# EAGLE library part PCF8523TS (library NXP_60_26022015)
The PCF8523 is a CMOS Real-Time Clock (RTC) and calendar optimized for low power consumption. Data is transferred serially via an I2C-bus with a maximum data rate of 1000 kbit/s. Alarm and timer functions are available with the possibility to generate a wake-up signal on an interrupt pin. An offset register allows fine-tuning of the clock. The PCF8523 has a backup battery switch-over circuit, which detects power failures and automatically switches to the battery supply when a power failure occurs. AAL Eindhoven MK
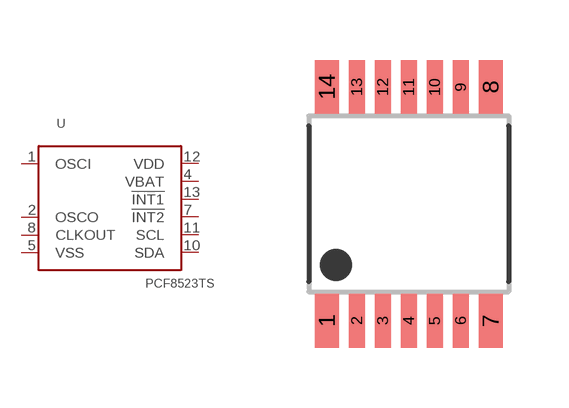
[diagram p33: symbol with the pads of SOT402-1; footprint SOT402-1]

Designator prefix -

## PCF8523TS  [SOT402-1]
1  OSCI  pas
2  OSCO  pas
4  VBAT  pwr
5  VSS  pwr
7  !INT2  out
8  CLKOUT  out
10  SDA
11  SCL  in
12  VDD  pwr
13  !INT1  out

## Footprint SOT402-1 (pad centres in mm)
SOT402-1 TSSOP14: plastic thin shrink small outline package; 14 leads; body width 4.4 mm JEDEC: MO-153 IEC: ---
smd 0.6 x 1.35: 1 -2.05,-2.925; 7 2.05,-2.925; 8 2.05,2.925; 14 -2.05,2.925
smd 0.4 x 1.35: 2 -1.3,-2.925; 3 -0.65,-2.925; 4 0,-2.925; 5 0.65,-2.925; 6 1.3,-2.925; 9 1.3,2.925; 10 0.65,2.925; 11 0,2.925; 12 -0.65,2.925; 13 -1.3,2.925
